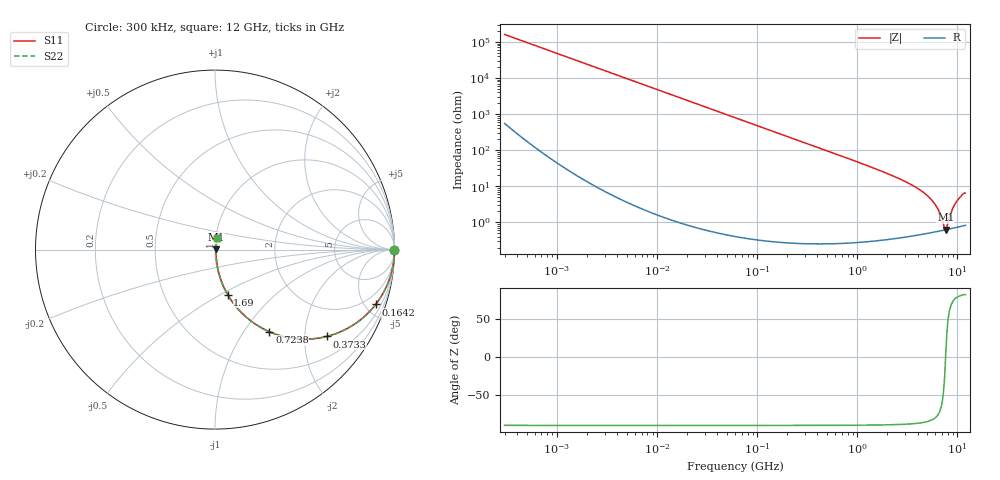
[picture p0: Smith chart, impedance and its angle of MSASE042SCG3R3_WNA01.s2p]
! MSASE042SCG3R3_WNA01  S-PARAMETER MODEL  ( General Type )
! Model Generated by TAIYO YUDEN Corporation (http://www.ty-top.com)
! Version 1.0
! TAIYO YUDEN Control No. 130801
! Copyright(c) 2013 TAIYO YUDEN CO.,LTD. All Rights Reserved.
! Product Description (link to TY-COMPAS)
! https://ds.yuden.co.jp/TYCOMPAS/or/detail?pn=MSASE042SCG3R3BWNA01&u=M
! Products Name : Multilayer Ceramic Capacitors
! Characteristics :
!  Capacitance : 3.3 pF , Rated Voltage : 16V , TCC : CG / C0G
!  Case Size : 0.4 x 0.2 / 0.016 x 0.008 [mm/inch] , Thickness : 0.2 / 0.008 [mm/inch]
!  (Conditions: Temperature = 25 degC , DC Bias Current/Voltage = 0A / 0V)
! External Node Assignments :
!  1  o---| |---o  2
! GND o---------o GND
! Frequency Range : 0.3MHz  -  12000MHz  [ 401 STEP ]
# MHz S RI R 50
! Freq[MHz].  S11 Real  S11 Imag  S21 Real  S21 Imag  S12 Real  S12 Imag  S22 Real  S22 Imag
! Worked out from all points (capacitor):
!   401 points, 300 kHz to 12 GHz, reference 50 ohm
!   read as one part in series: C = 3.31 pF near 316.3 kHz
!   lowest |Z| = 626 mohm at 7.649 GHz (marker M1)
!   series resonance near 7.613 GHz, so ESL is about 130 pH
!   S11 on the Smith chart (normalised r, x): 300 kHz: open; 164.2 MHz: 1.01, -5.85; 373.3 MHz: 1.01, -2.57; 723.8 MHz: 1.01, -1.32; 1.69 GHz: 1.01, -0.54; 12 GHz: 1.02, +0.13
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0.3  1 -0.000624  2.52e-06 0.000624  2.52e-06 0.000624  1 -0.000624
1.769972  1 -0.00368  1.58e-05 0.00368  1.58e-05 0.00368  1 -0.00368
10.44266  0.9995 -0.0217  0.000479 0.0217  0.000479 0.0217  0.9995 -0.0217
60  0.9846 -0.1229  0.0154 0.1229  0.0154 0.1229  0.9846 -0.1229
164.1901  0.8952 -0.3058  0.1048 0.3058  0.1048 0.3058  0.8952 -0.3058
353.9943  0.6472 -0.4769  0.3528 0.4769  0.3528 0.4769  0.6472 -0.4769
373.2558  0.6226 -0.4838  0.3774 0.4838  0.3774 0.4838  0.6226 -0.4838
723.8279  0.303 -0.4576  0.697 0.4576  0.697 0.4576  0.303 -0.4576
1076.992  0.1623 -0.3655  0.8377 0.3655  0.8377 0.3655  0.1623 -0.3655
1689.663  0.0707 -0.2506  0.9293 0.2506  0.9293 0.2506  0.0707 -0.2506
2088.533  0.0463 -0.2024  0.9537 0.2024  0.9537 0.2024  0.0463 -0.2024
3547.679  0.0152 -0.1041  0.9848 0.1041  0.9848 0.1041  0.0152 -0.1041
5006.236  0.00783 -0.0539  0.9922 0.0539  0.9922 0.0539  0.00783 -0.0539
6188.031  0.00618 -0.0262  0.9938 0.0262  0.9938 0.0262  0.00618 -0.0262
6699.894  0.006 -0.0161  0.994 0.0161  0.994 0.0161  0.006 -0.0161
7254.098  0.00604 -0.00617  0.994 0.00617  0.994 0.00617  0.00604 -0.00617
7648.807  0.00619 0.000618  0.9938 -0.000618  0.9938 -0.000618  0.00619 0.000618
8064.993  0.00644 0.00778  0.9936 -0.00778  0.9936 -0.00778  0.00644 0.00778
8732.115  0.00704 0.0185  0.993 -0.0185  0.993 -0.0185  0.00704 0.0185
9454.42  0.00801 0.0312  0.992 -0.0312  0.992 -0.0312  0.00801 0.0312
10793.46  0.0103 0.051  0.9897 -0.051  0.9897 -0.051  0.0103 0.051
12000  0.0122 0.0627  0.9878 -0.0627  0.9878 -0.0627  0.0122 0.0627
